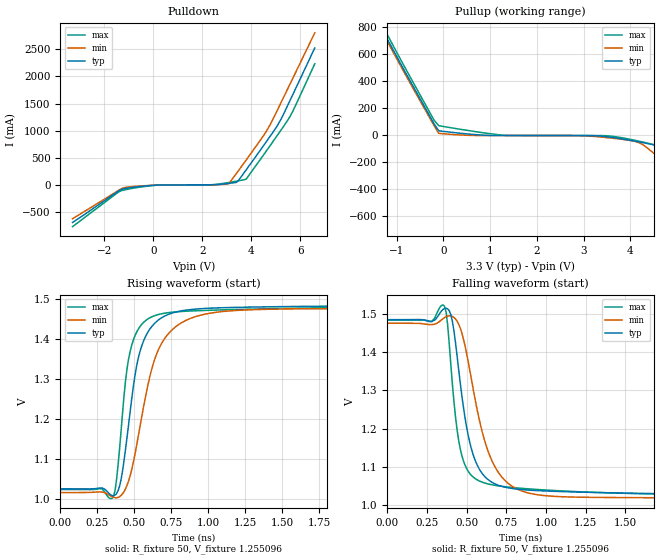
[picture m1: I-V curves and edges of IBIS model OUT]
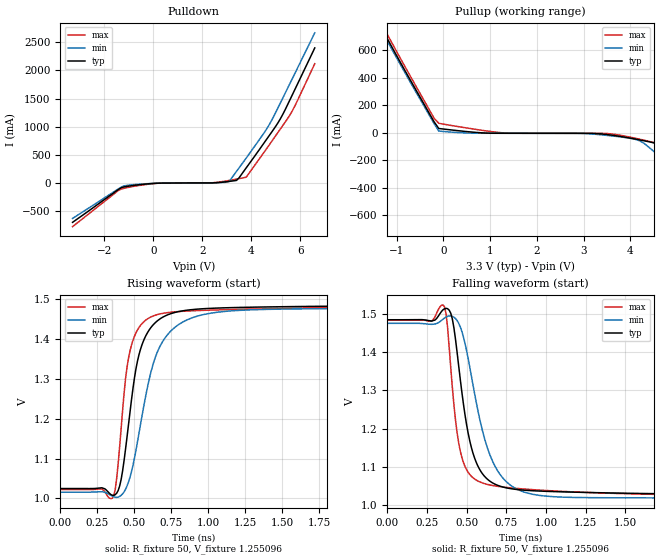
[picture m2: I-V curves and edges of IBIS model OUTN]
|   IBIS File of SG2520VGN C
|   LVDS, Vcc=3.3V, Io=4.5mA, fo>212.5MHz
[IBIS Ver]   3.2
[File Name]   sg2520vgn_hf_45m_33v.ibs
[File Rev]   1.0
[Date]   July 24, 2020
[Source]
Fairchild Ensigna Lab's Method
[Notes]
Created by Minoru Kozaki
[Disclaimer]
Seiko Epson Corporation makes no warranty with respect to the
information contained herein.
[Copyright]
Copyright(C) 2020, Seiko Epson Corporation. All rights reserved.
|   Component
[Component]   SG2520VGN
[Manufacturer]  Seiko Epson Corporation
[Package]
R_pkg   17.7m   NA   NA
L_pkg   235p   NA   NA
C_pkg   208f   NA   NA
[Pin]   signal_name   model_name   R_pin   L_pin   C_pin
1   OE/ST   NC
2   NC   NC
3   GND   GND
4   OUT   OUT   17.7m   235p   208f
5   OUTN   OUTN   10.4m   129p   221f
6   VCC   POWER
[Diff Pin] inv_pin  vdiff  tdelay_typ
4   5   0   0
| Models and submodels in the file (2): OUT (Output), OUTN (Output)
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|   Model OUT
[Model]   OUT
Model_type   Output
Polarity   Non-Inverting
Vref = 1.25
Vmeas = 1.25
Rref = 50
Cref = 0
C_comp   4.5p   4.5p   4.5p
[Temperature Range]   25   105   -40
[Voltage Range]   3.3   2.97   3.63
[Pullup Reference]   3.3   2.97   3.63
[Pulldown Reference]   0   0   0
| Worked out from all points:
|   slope of the pulldown table from 0 to 0.495 V, typ, clamps not added: 77.3 ohm
|   slope of the pullup table from 0 to 0.495 V, typ, clamps not added: 27 ohm
|   falling waveform, R_fixture 50, V_fixture 1.255096: 20-80 % time 115ps typ, 162ps min, 83.7ps max; typ from 1.49 V to 1.02 V
|   rising waveform, R_fixture 50, V_fixture 1.255096: 20-80 % time 122ps typ, 175ps min, 90.8ps max; typ from 1.02 V to 1.49 V
[Pullup]
-3.3V     2.52A      2.491A     2.553A
-1.4V     836.5mA    817mA      870.5mA
-1.3V     772.1mA    753.1mA    805.2mA
-1.2V     707.9mA    689.6mA    740.1mA
-200mV    81.95mA    68.77mA    108.4mA
-100mV    30.38mA    11.55mA    68.43mA
1.3V      -4.444mA   -4.554mA   -2.3mA
3.7V      -23.03mA   -27.2mA    -14.27mA
4.2V      -52.91mA   -59.14mA   -47.54mA
4.6V      -87.11mA   -163.3mA   -80.55mA
5.1V      -236.3mA   -303.9mA   -154.9mA
6.6V      -696.9mA   -716.6mA   -667.4mA
[Pulldown]
-3.3V     -686.5mA   -617.6mA   -762.2mA
-1.3V     -78.01mA   -65.02mA   -101.4mA
-900mV    -44.4mA    -28.37mA   -62.39mA
100mV     -755.3uA   -194.8uA   -2.605mA
2.3V      5.866mA    5.578mA    6.601mA
3.1V      32.86mA    32.76mA    49.64mA
3.4V      50.34mA    217.1mA    73.3mA
3.8V      283.7mA    464.3mA    111.9mA
4.6V      786.7mA    976.3mA    614.5mA
5.2V      1.197A     1.499A     1A
5.7V      1.663A     1.963A     1.357A
6.6V      2.524A     2.802A     2.232A
[Falling Waveform]
R_fixture = 50
V_fixture = 1.255096
V_fixture_min = 1.245192
V_fixture_max = 1.248643
0s        1.486V     1.476V     1.484V
360ps     1.515V     1.491V     1.521V
380ps     1.514V     1.495V     1.474V
410ps     1.482V     1.494V     1.318V
460ps     1.319V     1.463V     1.146V
530ps     1.147V     1.33V      1.077V
620ps     1.072V     1.159V     1.056V
750ps     1.045V     1.06V      1.047V
980ps     1.036V     1.025V     1.039V
4ns       1.025V     1.016V     1.023V
[Rising Waveform]
R_fixture = 50
V_fixture = 1.255096
V_fixture_min = 1.245192
V_fixture_max = 1.248643
0s        1.025V     1.016V     1.023V
360ps     1.008V     1.003V     1.008V
410ps     1.049V     1.008V     1.172V
440ps     1.125V     1.025V     1.296V
470ps     1.215V     1.057V     1.367V
540ps     1.372V     1.186V     1.432V
650ps     1.444V     1.363V     1.46V
800ps     1.469V     1.436V     1.468V
1.1ns     1.478V     1.469V     1.473V
4ns       1.485V     1.476V     1.484V
[Ramp]
R_load = 50
dV/dt_r   0.27723/123.15p   0.27675/174.49p   0.27446/86.70p
dV/dt_f   0.27723/115.03p   0.27675/163.35p   0.27446/85.81p
|   Model OUTN
[Model]   OUTN
Model_type   Output
Polarity   Inverting
Vref = 1.25
Vmeas = 1.25
Rref = 50
Cref = 0
C_comp   4.5p   4.5p   4.5p
[Temperature Range]   25   105   -40
[Voltage Range]   3.3   2.97   3.63
[Pullup Reference]   3.3   2.97   3.63
[Pulldown Reference]   0   0   0
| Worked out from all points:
|   slope of the pulldown table from 0 to 0.495 V, typ, clamps not added: 77.2 ohm
|   slope of the pullup table from 0 to 0.495 V, typ, clamps not added: 27.1 ohm
|   falling waveform, R_fixture 50, V_fixture 1.255096: 20-80 % time 113ps typ, 161ps min, 82.9ps max; typ from 1.49 V to 1.02 V
|   rising waveform, R_fixture 50, V_fixture 1.255096: 20-80 % time 122ps typ, 173ps min, 89.6ps max; typ from 1.02 V to 1.49 V
[Pullup]
-3.3V     2.395A     2.371A     2.423A
-1.4V     807.5mA    788.5mA    840.4mA
-1.3V     745.4mA    726.9mA    777.4mA
-1.2V     683.4mA    665.7mA    714.5mA
-200mV    79.29mA    66.45mA    105.1mA
-100mV    30.32mA    11.54mA    68.22mA
1.3V      -4.444mA   -4.554mA   -2.303mA
3.7V      -23.07mA   -27.28mA   -14.29mA
4.2V      -53.04mA   -59.33mA   -47.69mA
4.6V      -87.2mA    -164.3mA   -80.83mA
5.1V      -237.5mA   -306.1mA   -154.4mA
6.6V      -702.5mA   -723.3mA   -672mA
[Pulldown]
-3.3V     -692.5mA   -623.5mA   -768mA
-1.3V     -78.17mA   -65.3mA    -101.5mA
-900mV    -44.47mA   -28.46mA   -62.53mA
100mV     -758.4uA   -196.6uA   -2.612mA
2.3V      5.867mA    5.579mA    6.604mA
3.1V      32.79mA    31.77mA    49.48mA
3.4V      50.21mA    209.7mA    73.04mA
3.8V      274.1mA    448.3mA    108.6mA
4.7V      821.1mA    1.009A     655.3mA
5.2V      1.147A     1.428A     965.8mA
5.7V      1.583A     1.869A     1.297A
6.6V      2.399A     2.666A     2.119A
[Falling Waveform]
R_fixture = 50
V_fixture = 1.255096
V_fixture_min = 1.245192
V_fixture_max = 1.248643
0s        1.485V     1.476V     1.484V
350ps     1.511V     1.487V     1.524V
390ps     1.511V     1.496V     1.414V
430ps     1.434V     1.489V     1.222V
470ps     1.296V     1.455V     1.124V
530ps     1.15V      1.338V     1.075V
620ps     1.071V     1.164V     1.055V
750ps     1.044V     1.061V     1.045V
980ps     1.036V     1.023V     1.038V
4ns       1.025V     1.016V     1.023V
[Rising Waveform]
R_fixture = 50
V_fixture = 1.255096
V_fixture_min = 1.245192
V_fixture_max = 1.248643
0s        1.025V     1.015V     1.022V
360ps     1.008V     1.004V     1.007V
410ps     1.047V     1.008V     1.175V
440ps     1.124V     1.023V     1.301V
470ps     1.217V     1.053V     1.37V
540ps     1.373V     1.184V     1.433V
650ps     1.444V     1.363V     1.46V
800ps     1.469V     1.436V     1.469V
1.1ns     1.478V     1.468V     1.473V
4ns       1.485V     1.476V     1.484V
[Ramp]
R_load = 50
dV/dt_r   0.27694/122.03p   0.27647/172.08p   0.27417/85.29p
dV/dt_f   0.27694/113.71p   0.27647/162.04p   0.27417/84.21p
